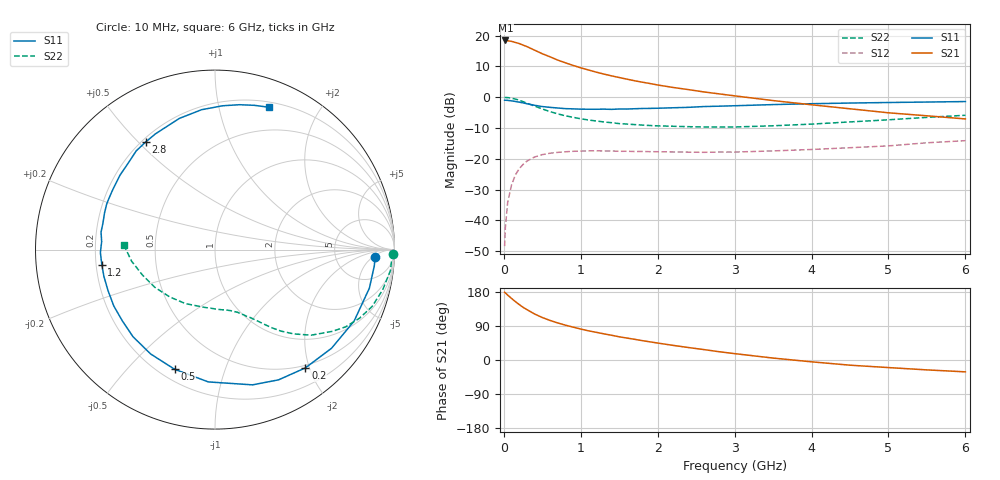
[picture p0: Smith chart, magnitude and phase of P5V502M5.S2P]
! SIEMENS Small Signal Semiconductors
! BFP183
! Si NPN RF Bipolar Junction Transistor in SOT143
! VCE = 0.5 V  IC = 2.5 mA
! Common Emitter S-Parameters:  March  1996
# GHz  S  MA  R  50
!  f  S11  S21  S12  S22
! GHz  MAG  ANG  MAG  ANG  MAG  ANG  MAG  ANG
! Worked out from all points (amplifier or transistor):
!   36 points, 10 MHz to 6 GHz, reference 50 ohm
!   highest |S21| = 18.4 dB at 20 MHz (marker M1)
!   |S21| within 3 dB of that: start of sweep to 386.4 MHz
!   unconditionally stable (mu >= 1): 1.811 GHz to end of sweep
!   at 250 MHz: K = 0.16, MSG = 19.4 dB, |S12| = -21.8 dB
!   at 1.4 GHz: K = 0.80, MSG = 12.2 dB, |S12| = -17.5 dB
!   at 6 GHz: K = 1.23, MAG = 0.7 dB, |S12| = -14.1 dB
!   S11 on the Smith chart (normalised r, x): 10 MHz: 15, -6; 200 MHz: 0.46, -1.94; 500 MHz: 0.26, -0.68; 1.2 GHz: 0.22, -0.06; 2.8 GHz: 0.22, +0.53; 6 GHz: 0.25, +1.42
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0.01  0.893 -2.7  8.32 178.6  0.0038 89.2  0.9937 -1.3
0.02  0.8922 -5.8  8.335 177.0  0.0077 85.1  0.9865 -2.7
0.05  0.8866 -14.0  8.248 171.2  0.0196 83.6  0.9846 -6.8
0.1  0.8713 -27.2  8.057 162.5  0.0374 74.6  0.9607 -13.5
0.15  0.8508 -40.2  7.733 154.1  0.0546 67.5  0.9309 -19.9
0.2  0.8295 -52.6  7.427 146.3  0.0688 60.8  0.8912 -25.4
0.25  0.8074 -64.0  7.011 139.0  0.081 54.8  0.8455 -30.6
0.3  0.782 -74.5  6.626 133.0  0.0915 49.9  0.7976 -34.8
0.4  0.7381 -92.9  5.794 121.3  0.1067 41.2  0.7167 -41.7
0.5  0.7036 -108.7  5.07 112.1  0.1166 34.5  0.6435 -46.9
0.6  0.6831 -121.7  4.523 104.4  0.1228 29.1  0.5831 -51.1
0.7  0.6665 -133.3  4.002 97.8  0.1268 24.9  0.5352 -54.2
0.8  0.651 -142.7  3.615 91.9  0.1296 21.4  0.4982 -56.6
1.1  0.6368 -166.4  2.766 77.0  0.1341 14.2  0.4256 -62.7
1.2  0.6362 -172.5  2.551 73.1  0.1344 12.0  0.4103 -64.8
1.7  0.6485 161.6  1.847 54.6  0.131 7.2  0.3584 -73.7
2.2  0.6723 142.0  1.437 38.6  0.129 5.5  0.3367 -84.1
2.8  0.7136 122.6  1.13 21.8  0.1283 6.6  0.3271 -99.1
3.5  0.7574 105.2  0.88 5.1  0.134 8.7  0.3429 -118.6
4.5  0.8024 87.0  0.647 -13.7  0.1509 10.1  0.3962 -148.1
5.5  0.833 74.8  0.498 -26.1  0.1815 9.3  0.4696 -172.2
6  0.8483 69.2  0.443 -31.3  0.1965 6.1  0.5081 177.2
